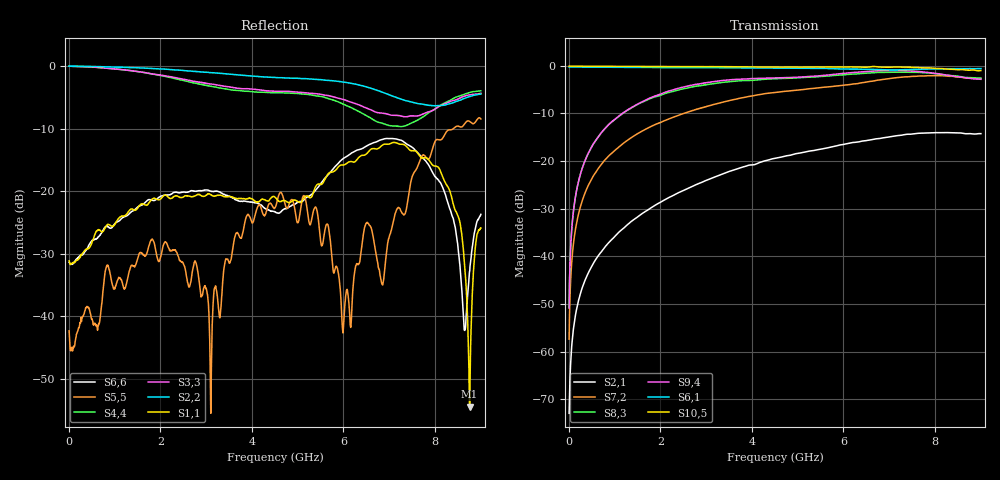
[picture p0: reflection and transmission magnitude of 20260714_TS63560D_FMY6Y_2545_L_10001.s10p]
# GHz S DB R 50
! CMT, SN0916, 25263762, 26.7.0
! Date: 15.07.2026 13:41:51
! Data: Format
! Freq S1.1:dB/Ang S1.2:dB/Ang S1.3:dB/Ang S1.4:dB/Ang S1.5:dB/Ang S1.6:dB/Ang S1.7:dB/Ang S1.8:dB/Ang S1.9:dB/Ang S1.10:dB/Ang
!  S2.1:dB/Ang S2.2:dB/Ang S2.3:dB/Ang S2.4:dB/Ang S2.5:dB/Ang S2.6:dB/Ang S2.7:dB/Ang S2.8:dB/Ang S2.9:dB/Ang S2.10:dB/Ang
!  S3.1:dB/Ang S3.2:dB/Ang S3.3:dB/Ang S3.4:dB/Ang S3.5:dB/Ang S3.6:dB/Ang S3.7:dB/Ang S3.8:dB/Ang S3.9:dB/Ang S3.10:dB/Ang
!  S4.1:dB/Ang S4.2:dB/Ang S4.3:dB/Ang S4.4:dB/Ang S4.5:dB/Ang S4.6:dB/Ang S4.7:dB/Ang S4.8:dB/Ang S4.9:dB/Ang S4.10:dB/Ang
!  S5.1:dB/Ang S5.2:dB/Ang S5.3:dB/Ang S5.4:dB/Ang S5.5:dB/Ang S5.6:dB/Ang S5.7:dB/Ang S5.8:dB/Ang S5.9:dB/Ang S5.10:dB/Ang
!  S6.1:dB/Ang S6.2:dB/Ang S6.3:dB/Ang S6.4:dB/Ang S6.5:dB/Ang S6.6:dB/Ang S6.7:dB/Ang S6.8:dB/Ang S6.9:dB/Ang S6.10:dB/Ang
!  S7.1:dB/Ang S7.2:dB/Ang S7.3:dB/Ang S7.4:dB/Ang S7.5:dB/Ang S7.6:dB/Ang S7.7:dB/Ang S7.8:dB/Ang S7.9:dB/Ang S7.10:dB/Ang
!  S8.1:dB/Ang S8.2:dB/Ang S8.3:dB/Ang S8.4:dB/Ang S8.5:dB/Ang S8.6:dB/Ang S8.7:dB/Ang S8.8:dB/Ang S8.9:dB/Ang S8.10:dB/Ang
!  S9.1:dB/Ang S9.2:dB/Ang S9.3:dB/Ang S9.4:dB/Ang S9.5:dB/Ang S9.6:dB/Ang S9.7:dB/Ang S9.8:dB/Ang S9.9:dB/Ang S9.10:dB/Ang
!  S10.1:dB/Ang S10.2:dB/Ang S10.3:dB/Ang S10.4:dB/Ang S10.5:dB/Ang S10.6:dB/Ang S10.7:dB/Ang S10.8:dB/Ang S10.9:dB/Ang S10.10:dB/Ang
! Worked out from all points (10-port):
!   2001 points, 10 MHz to 9 GHz, reference 50 ohm
!   strongest paths, dB at 10 MHz, 2.257 GHz, 4.505 GHz, 6.753 GHz, 9 GHz:
!     S10,5: -0.1, -0.2, -0.2, -0.2, -1.0
!     S6,1: -0.2, -0.4, -0.5, -0.8, -0.6
!     S9,4: -50.8, -5.1, -2.5, -1.0, -2.8
!     S8,3: -50.7, -5.4, -2.7, -1.4, -2.6
!     S7,2: -57.4, -10.9, -5.6, -3.0, -2.7
!     S2,1: -73.0, -27.3, -19.4, -15.3, -14.2
!   lowest |S11| = -54.4 dB at 8.753 GHz (marker M1), VSWR 1.00, Z = 50 - j0.19 ohm
!   |S11| at or under -10 dB: start of sweep to end of sweep
